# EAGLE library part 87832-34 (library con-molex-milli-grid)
HEADER
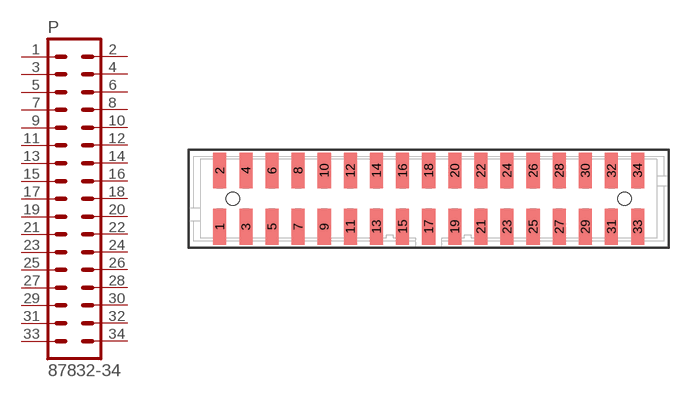
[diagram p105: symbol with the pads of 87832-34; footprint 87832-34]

Designator prefix P

## 87832-34  [87832-34]
1  1  pas
2  2  pas
3  3  pas
4  4  pas
5  5  pas
6  6  pas
7  7  pas
8  8  pas
9  9  pas
10  10  pas
11  11  pas
12  12  pas
13  13  pas
14  14  pas
15  15  pas
16  16  pas
17  17  pas
18  18  pas
19  19  pas
20  20  pas
21  21  pas
22  22  pas
23  23  pas
24  24  pas
25  25  pas
26  26  pas
27  27  pas
28  28  pas
29  29  pas
30  30  pas
31  31  pas
32  32  pas
33  33  pas
34  34  pas

## Footprint 87832-34 (pad centres in mm)
HEADER SMD Dual Row, Shrouded, Vertical
smd 1 x 2.75: 1 -16,-2.15; 2 -16,2.15; 3 -14,-2.15; 4 -14,2.15; 5 -12,-2.15; 6 -12,2.15; 7 -10,-2.15; 8 -10,2.15; 9 -8,-2.15; 10 -8,2.15; 11 -6,-2.15; 12 -6,2.15; 13 -4,-2.15; 14 -4,2.15; 15 -2,-2.15; 16 -2,2.15; 17 0,-2.15; 18 0,2.15; 19 2,-2.15; 20 2,2.15; 21 4,-2.15; 22 4,2.15; 23 6,-2.15; 24 6,2.15; 25 8,-2.15; 26 8,2.15; 27 10,-2.15; 28 10,2.15; 29 12,-2.15; 30 12,2.15; 31 14,-2.15; 32 14,2.15; 33 16,-2.15; 34 16,2.15
hole 1 at -15,0
hole 1 at 15,0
